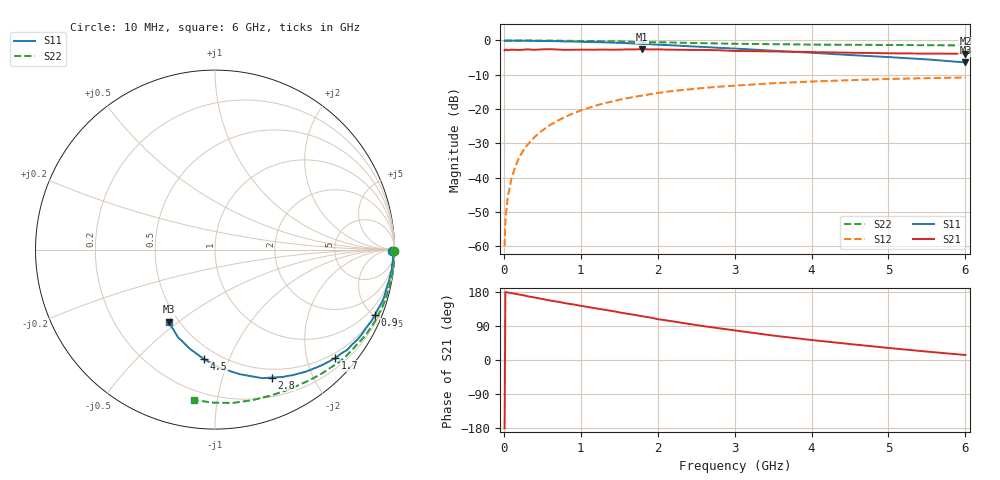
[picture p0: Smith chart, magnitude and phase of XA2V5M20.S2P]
! SIEMENS Discrete & RF Semiconductors
! BFY180
! Si NPN RF Bipolar Junction Transistor in MICRO-X
! VCE = 2.5 V  IC = 0.2 mA
! Common Emitter S-Parameters:  May  1997
# GHz  S  MA  R  50
!  f  S11  S21  S12  S22
! GHz  MAG  ANG  MAG  ANG  MAG  ANG  MAG  ANG
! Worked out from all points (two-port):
!   36 points, 10 MHz to 6 GHz, reference 50 ohm
!   highest |S21| = -2.55 dB at 1.8 GHz (marker M1); lowest = -3.9 dB at 6 GHz (marker M2)
!   |S21| within 3 dB of the highest: start of sweep to end of sweep
!   lowest |S11| = -6.4 dB at 6 GHz (marker M3), VSWR 2.83, Z = 22.1 - j23 ohm
!   |S11| at or under -10 dB: nowhere
!   |S22| runs from -1.5 to 0.0 dB; largest |S21 - S12| = 0.74
!   S11 on the Smith chart (normalised r, x): 10 MHz: open; 900 MHz: 0.49, -5.03; 1.7 GHz: 0.39, -2.55; 2.8 GHz: 0.40, -1.46; 4.5 GHz: 0.42, -0.81; 6 GHz: 0.44, -0.46
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0.01  0.9886 -0.3  0.715 -180.0  0.001 87.5  0.9995 -0.3
0.02  0.9974 -0.5  0.739 179.2  0.0024 96.3  0.9999 -0.4
0.05  0.9939 -1.1  0.721 178.1  0.0052 90.0  0.9991 -1.0
0.1  0.9927 -2.6  0.735 176.5  0.0097 88.8  0.9994 -2.1
0.15  0.9938 -3.9  0.73 174.6  0.0146 87.3  0.9999 -3.0
0.2  0.9892 -5.0  0.727 172.8  0.0197 85.4  0.9987 -4.0
0.3  0.9884 -7.3  0.742 168.6  0.0294 83.8  0.9981 -6.0
0.4  0.9852 -10.0  0.731 164.9  0.0392 81.5  0.9981 -8.0
0.5  0.9801 -12.5  0.742 161.0  0.0487 78.9  0.9953 -10.0
0.7  0.9755 -17.4  0.737 153.8  0.0676 74.5  0.9915 -14.0
0.9  0.9636 -22.3  0.732 146.7  0.0864 70.4  0.9866 -18.0
1.1  0.9485 -27.2  0.734 139.6  0.1036 66.1  0.9791 -21.9
1.3  0.9386 -32.3  0.736 132.8  0.1209 61.6  0.9726 -25.9
1.7  0.9029 -42.0  0.74 119.2  0.1503 53.7  0.9518 -33.4
1.8  0.8897 -44.5  0.746 115.3  0.1577 52.0  0.9486 -35.2
2.2  0.8479 -53.3  0.733 101.8  0.1834 44.1  0.9334 -42.3
2.8  0.7798 -66.1  0.719 83.7  0.2119 34.0  0.9039 -51.9
3.5  0.7086 -78.6  0.692 64.5  0.2376 24.0  0.882 -62.0
4  0.661 -87.4  0.677 52.8  0.2515 17.2  0.8705 -69.2
4.5  0.6131 -95.8  0.663 42.1  0.2637 11.1  0.8641 -76.2
5.5  0.5296 -113.0  0.643 22.2  0.2818 -0.7  0.8529 -90.6
6  0.4779 -122.7  0.641 13.1  0.2882 -6.7  0.8458 -97.8
